FUNCTION_BLOCK FB 15
TITLE = FactoryLink S7 Read
// KNOW_HOW_PROTECT
AUTHOR : DLink
FAMILY : SAPI_S7
NAME   : S7_READ
VERSION: 1.0


VAR_INPUT
  ID      : WORD;                      // Connection number, taken from CO configuration
END_VAR

VAR_OUTPUT
  DONE    : BOOL;                      // True if no error from AG-SEND/RECV
  ERROR   : BOOL;                      // True if any error from AG-SEND/RECV
  STATUS  : WORD;                      // Error status from AG-RECV
END_VAR

VAR
  R_NDR   : BOOL;                      // Set when data retrieved
  R_ERROR : BOOL;                      // Set when there was an error by AG-RECV
  S_DONE  : BOOL;                      // Set when there AG-SEND completes a frame
  S_ERROR : BOOL;                      // Set when AG-SEND has an error
  S_ACT   : BOOL;                      // Trigger to send a new frame with AG-SEND
  Sending : BOOL;                      // Indicates that we are sending data
  R_LEN   : WORD;                      // Received no. of bytes
  S_LEN   : WORD;                      // No of bytes to send to partner

  Recv_Buf: STRUCT                     // Buffer to receive "Fetch" request
   Sys_ID   : WORD;                    // Must contain 'S7' chars
   Opcod1   : WORD;                    // Must contain the value b#(16,01)
   Opcod2   : WORD;                    // Must contain the value b#(03,05)
   Opcod3   : WORD;                    // Must contain the value b#(03,08)
   Org_ID   : BYTE;                    // Must contain the value 01 = DB request
   DB_No    : BYTE;                    // The requested DB no. 1-255
   DW_No    : WORD;                    // The start offset = Start DW no. 0-2047
   Len      : WORD;                    // No of words to send back. 1-112 are allowed for CP443/343
   End_blck : WORD;                    // End header info. must contain B#(255,02)
  END_STRUCT ;

  Send_Buf: STRUCT                     // Send buffer for fetch request
   Sys_ID   : WORD := W#16#5337;       // Must contain 'S7' chars
   Opcod1   : WORD := W#16#1001;       // Must contain the value b#(16,01)
   Opcod2   : WORD := W#16#306;        // Must contain the value b#(03,06)
   Opcod3   : WORD := W#16#F03;        // Must contain the value b#(0f,03)
   Err_No   : BYTE;                    // Contains either 0 = OK or errorcode
   Emp_Blck : BYTE := B#16#FF;         // Always xff, Indicating empty block
   Emp_Len  : BYTE := B#16#7;          // Lenght of unused header info
   DispHead1: WORD;                    // Not used part of header
   DispHead2: WORD;                    // Not used part of header
   Data     : ARRAY [0..8192] OF BYTE; // Real data to send to the partner (112 words)
  END_STRUCT ;

  BSEND    : SFB 12;     // Local instance of SFB 12

  BRECV    : SFB 13;  // Local instance of SFB 13

END_VAR

VAR_TEMP
  Source_Ptr: ANY;                     // Pointer to the target Data in this PLC's DB
  Dest_Ptr  : ANY;                     // Pointer to the internal data buf with user data
  Recv_Ptr  : ANY;                     // Pointer to the recv area in this instance DB
  Send_Ptr  : ANY;                     // Pointer to send area in this instance DB
  EN_STATUS : BOOL;                    // used only for EN, ENO operation
  Int_Var   : INT;                     // Temporary integer value
  Max_Adr   : DWORD;                   // Maximum allowed address
  DB_Offset : WORD;                    // DB Number offset for nr. > 255
  LADDR     : DWORD;                   // CP module logical Baseaddress, from System Configuration
  S5        : BOOL;                    // S5 Addressing mode, when true
END_VAR

BEGIN
NETWORK
TITLE =

      SET   ;
      SAVE  ;
      =     #EN_STATUS;                // save if any uses the EN, ENO status
      SET   ;                          // Make sure all info bits are zero
      R     #R_NDR;
      R     #S_DONE;
      R     #R_ERROR;
      R     #S_ERROR;
      R     #S_ACT;
      R     #S5;
      L     0;                         // Reset error code
      T     #STATUS;
      L     1;                         // remote id
      T     #LADDR;

//
// Prepare the needed ANY pointers, so most of the initialization are done now.
// Cannot use static area for ANY pointers, must use local variable and build them up
//
      L     W#16#1002;                 // S7 syntax ID and lentype = 10 hex and 04 (words)
      T     LW     0;                  // Begin Create ANY WORD Ptr, here SourcePtr
      T     LW    10;                  // DestPtr
      L     W#16#1002;                 // This is a type BYTE = 02
      T     LW    20;                  // Pointer to our local receivebuffer
      T     LW    30;                  // Pointer to our local send buffer
      L     224;                       // This is in bytess, because we have a byte ptr
      T     LW    12;                  // Max len for Dest Ptr
      L     16;                        // Lenght of receive buffer (max)
      T     LW    22;                  // to Recv_ptr
      L     240;                       // Lenght of send buffer including the header
      T     LW    32;                  // to Send_Ptr
      L     DINO;                      // our own instance DB no
      T     LW    14;                  // DestPtr is always in our own DB
// 	L 	13;				   // Load DB 13
      T     LW    24;                  // Recv_Ptr Too
// 	L 	12;				   // Load DB 12
      T     LW    34;                  // Same with Send_ptr
      L     W#16#8400;                 // DB area type pointer
      T     LW     6;                  // Are the same for all pointers
      T     LW    16;                  // set dest ptr
      T     LW    26;                  // set recv ptr
      T     LW    36;                  // set send ptr
      L     12;                        // start offset for recv_buf
      SLW   3;
      T     LW    28;                  // set for recv_ptr
      L     28;                        // start offset send_ptr
      SLW   3;
      T     LW    38;                  // set for send_ptr
      L     16;
      T     #S_LEN;
//
// See If there is anything to receive from a partner (a request)
//
      CALL  sfb 13,db13(
            EN_R   := TRUE,
            ID     := #ID,             // Connection ID from CO config.
            R_ID   := W#16#1,          // Module base adr. from System Config.
            NDR    := #R_NDR,          // Set if data received
            ERROR  := #R_ERROR,        // Set if there was an error
            STATUS := #STATUS,         // Receive status information
            RD_1   := #Recv_Ptr,       // Our newly build ANY pointer to our own DB
            LEN    := #R_LEN);         // No of databytes received


      A     #Sending;                  // May not receive, while sending
      JC    SKIP;
//
// Anything received ??
//

      A     #R_ERROR;
      JC    NERR;
      AN    #R_NDR;
      JC    NERR;                      // skip if not
      L     0;                         // reset addressing above 255
      T     #DB_Offset;
      L     16;
      L     #R_LEN;                    // Received exactly 16 bytes
      <>I   ;
      JC    ERR1;
      L     'S7';                      // This must be the in first 2 bytes
      L     #Recv_Buf.Sys_ID;
      <>I   ;
      JC    ERR1;
      L     W#16#1001;                 // must contain this value
      L     #Recv_Buf.Opcod1;
      <>I   ;
      JC    ERR1;
      L     W#16#305;                  // and this
      L     #Recv_Buf.Opcod2;
      <>I   ;
      JC    ERR1;
      L     W#16#308;                  // and this
      L     #Recv_Buf.Opcod3;
      <>I   ;
      JC    ERR1;
      L     W#16#FF02;                 // and this too
      L     #Recv_Buf.End_blck;
      <>I   ;
      JC    ERR1;
      L     1;
      L     #Recv_Buf.Org_ID;          // We expect only DB, FB IB and QB indentifier
      >I    ;
      JC    ERR2;                      // Send a header with error-info to our partner
      L     4;
      <=I   ;
      JC    EVAL;                      // Normal addressing parameters
      L     120;                       // Check for addressing above 255
      L     #Recv_Buf.Org_ID;
      >I    ;
      JC    ERR2;                      // Send a header with error-info to our partner
      L     134;
      >I    ;
      JC    ERR2;                      // Check for flagbytes above 255
      L     #Recv_Buf.Org_ID;          // Remove offset of 20
      L     119;
      -I    ;                          // Number of blocks
      L     256;                       // Block size of 256
      *I    ;                          // Offset
      T     #DB_Offset;                 // Activate offset
      L     1;
      T     #Recv_Buf.Org_ID;          // Adjust org id to normal value
//
// Evaluate received identifier
//
EVAL: L     1;
      L     #Recv_Buf.Org_ID;          // Evaluat DB indentifier
      <I    ;
      JC    I_FB;
      AN    #S5;                       // Check for word boundary
      JC    I_DB;
      L     #Recv_Buf.DW_No;           // Start address is to be doubled
      SLW   1;
      T     #Recv_Buf.DW_No;
      L     #Recv_Buf.Len;             // Length is to be doubled
      SLW   1;
      T     #Recv_Buf.Len;
I_DB: L     L#+65534;                  // Max. address
      T     #Max_Adr;
      JU    ADDR;                      // Go check address
I_FB: L     0;                         // Not a DB so set DBNR to zero
      T     #Recv_Buf.DB_No;
      L     2;
      L     #Recv_Buf.Org_ID;          // Evaluat FB indentifier
      <I    ;
      JC    I_IB;
      L     W#16#8300;                 // FB area type pointer
      T     LW     6;
      L     L#+2047;                   // Max. address
      T     #Max_Adr;
      JU    ADDR;                      // Go check address
I_IB: L     3;
      L     #Recv_Buf.Org_ID;          // Evaluat FB indentifier
      <I    ;
      JC    I_QB;
      L     W#16#8100;                 // IB area type pointer
      T     LW     6;
      L     L#+8191;                   // Max. address
      T     #Max_Adr;
      JU    ADDR;                      // Go check address
I_QB: L     W#16#8200;                 // QB area type pointer
      T     LW     6;
      L     L#+8191;                   // Max. address
      T     #Max_Adr;
ADDR: L     #Max_Adr;                  // Check begin address
      L     #Recv_Buf.DW_No;           // Must be =< 2047
      <D    ;
      JC    ERR2;                      //
      L     0;
      L     #Recv_Buf.Len;             // Must be 1..112 datawords (224 bytes max)
      >=I   ;
      JC    ERR2;                      //
      L     8192;
      >I    ;
      JC    ERR2;
      L     #Recv_Buf.Len;
      L     #Recv_Buf.DW_No;
      +I    ;                          // Calculate the end addres
      +     -1;
      L     #Max_Adr;                  // Compare with max. address
      >D    ;
      JC    ERR2;
//
// Copy from local DB to our own instance DB's Sendbuffer
//
      L     44;                        // Start offset for Dest_ptr = Data[0]
      SLW   3;
      T     LW    18;                  // Now set for Dest Ptr
      L     #Recv_Buf.Len;             // No. of words
      T     LW     2;                  // Max words to pointer
      +     16;
      T     #S_LEN;                    // may be changed later
      L     #Recv_Buf.DB_No;           // Get target DB
      L     #DB_Offset;
      +I    ;
      T     LW     4;                  // To source ptr
      L     #Recv_Buf.DW_No;           // Get target DW
      SLD   3;                         // Adjust for Words and Pointer
      T     LW     8;                  // To source ptr
      SRD   16;                        // Save first three bits
      L     7;
      AW    ;                          // Remove not used bits
      T     LB     7;
//
// Block move
//
      CALL  SFC   20 (
            SRCBLK  := #Source_Ptr,
            RET_VAL := #Int_Var,
            DSTBLK  := #Dest_Ptr);

      L     #Int_Var;                  // Get result from the block move
      L     0;                         // Should be Zero if OK.
      T     #Send_Buf.Err_No;          // In case there is no error
      ==I   ;
      JC    CONT;                      // Ok Continue if every thing is fine
      S     R_ERROR;
      L     #Int_Var;
      T     #STATUS;
ERR3: L     4;                         // Block move error
      T     #Send_Buf.Err_No;
      L     16;
      T     #S_LEN;
      JU    CONT;
ERR2: L     3;                         // This is the same as send from a S5 PLC
      T     #Send_Buf.Err_No;
      L     16;
      T     #S_LEN;
      JU    CONT;
ERR1: L     5;                         // This is the same as send from a S5 PLC
      T     #Send_Buf.Err_No;
      L     16;
      T     #S_LEN;
      JU    CONT;

//
// Create the H1 Fetch reply header information to make sure it is set up
//
CONT: L     'S7';
      T     #Send_Buf.Sys_ID;
      L     W#16#1001;
      T     #Send_Buf.Opcod1;
      L     W#16#306;
      T     #Send_Buf.Opcod2;
      L     W#16#F03;
      T     #Send_Buf.Opcod3;
      L     B#16#FF;
      T     #Send_Buf.Emp_Blck;
      L     B#16#7;
      T     #Send_Buf.Emp_Len;
      SET   ;
      =     #S_ACT;
      S     #Sending;
SKIP: NOP   0;
//
// Send the requested data to the active partner
//
      L     1;                         // remote id
      T     #LADDR;
      CALL  sfb 12, db12 (
            REQ    := #S_ACT,
            R      := FALSE,
            ID     := #ID,
            R_ID   := #LADDR,
            DONE   := #S_DONE,
            ERROR  := #S_ERROR,
            STATUS := #STATUS,
            SD_1   := #Send_Ptr,
            LEN    := #S_LEN);
//
// The send function returns with a unknown error kode H7000
// after completing a sendjob or when not doing anything
// For now we just shortcircuit this problem but it must be solved by Siemens
//
      L     #STATUS;                   // Get send status
      L     W#16#7000;                 // Not Know error status
      <>I   ;                          // skip if not unknown status
      JC    NERR;
      L     W#16#8181;                 // force default status
      T     #STATUS;                   // Into the status info
      A     #S_ERROR;                  // and clear the error indikation
      R     #S_ERROR;
      R     #Sending;
//
// Final work before exit from this function
//
NERR: A     #S_DONE;                   // Sending completed
      =     #DONE;                     // Mark done flag
      A     #S_DONE;                   // Enable Reception after job completed or
      O     #S_ERROR;                  // there was an error
      R     #Sending;
      O     #R_ERROR;                  // error indication on either AG-RECV or AG-SEND
      O     #S_ERROR;
      AN    #S_DONE;
      =     #ERROR;                    // are send out
      CLR;                             // restore the EN status to ENO
      A     #EN_STATUS;
      SAVE;
END_FUNCTION_BLOCK
